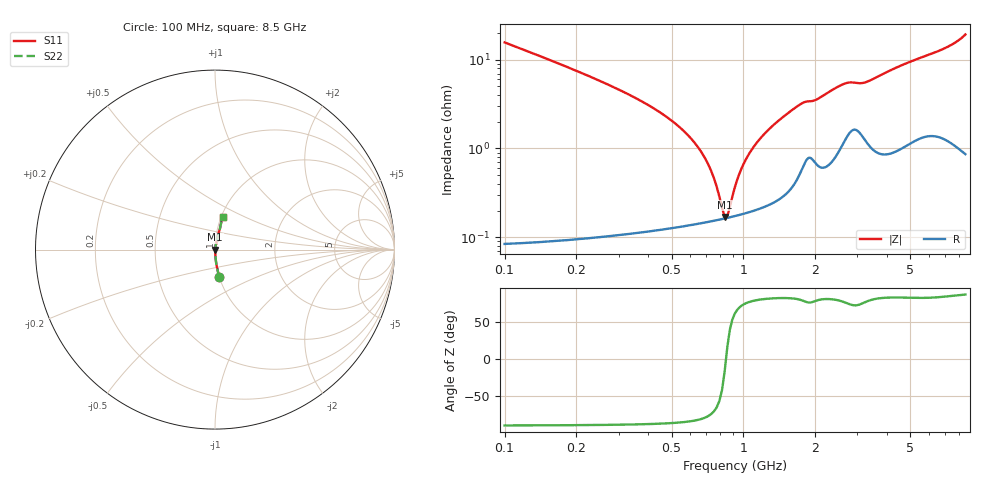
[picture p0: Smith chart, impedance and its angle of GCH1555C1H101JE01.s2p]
!Murata Part Number: GCH1555C1H101JE01
!These Parameters are Measured in Series Mode Connection
!Data Generated on Jun 19, 2026
!  o--ll--o
!Port1  Port2
!  o------o
!Operation Temp=25[degC], DC Bias Voltage=0[V]
!Freq. Start=100[MHz] Stop=9[GHz] 401[Steps]
# Hz S RI R 50
!Freq.(Hz) S11(Real) S11(Imag) S21(Real) S21(Imag) S12(Real) S12(Imag) S22(Real) S22(Imag)
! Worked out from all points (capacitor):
!   401 points, 100 MHz to 8.5 GHz, reference 50 ohm
!   read as one part in series: C = 100 pF near 142 MHz
!   lowest |Z| = 169 mohm at 835 MHz (marker M1)
!   series resonance near 845.3 MHz, so ESL is about 350 pH
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1e8  0.0248 -0.1528  0.9752 0.1528  0.9752 0.1528  0.0248 -0.1528
2.47e8  0.00443 -0.0585  0.9956 0.0585  0.9956 0.0585  0.00443 -0.0585
5.41e8  0.0016 -0.0172  0.9984 0.0172  0.9984 0.0172  0.0016 -0.0172
6.46e8  0.00152 -0.0102  0.9985 0.0102  0.9985 0.0102  0.00152 -0.0102
7.09e8  0.00153 -0.00661  0.9985 0.00661  0.9985 0.00661  0.00153 -0.00661
8.14e8  0.0016 -0.00141  0.9984 0.00141  0.9984 0.00141  0.0016 -0.00141
8.35e8  0.00163 -0.000457  0.9984 0.000457  0.9984 0.000457  0.00163 -0.000457
8.56e8  0.00165 0.000475  0.9984 -0.000475  0.9984 -0.000475  0.00165 0.000475
8.77e8  0.00168 0.00138  0.9983 -0.00138  0.9983 -0.00138  0.00168 0.00138
9.82e8  0.00184 0.00566  0.9982 -0.00566  0.9982 -0.00566  0.00184 0.00566
1.087e9  0.00205 0.0096  0.998 -0.0096  0.998 -0.0096  0.00205 0.0096
1.255e9  0.00249 0.0154  0.9975 -0.0154  0.9975 -0.0154  0.00249 0.0154
1.507e9  0.00362 0.0237  0.9964 -0.0237  0.9964 -0.0237  0.00362 0.0237
1.759e9  0.00681 0.0314  0.9932 -0.0314  0.9932 -0.0314  0.00681 0.0314
2.011e9  0.00789 0.0342  0.9921 -0.0342  0.9921 -0.0342  0.00789 0.0342
2.473e9  0.0109 0.0476  0.9891 -0.0476  0.9891 -0.0476  0.0109 0.0476
2.914e9  0.0187 0.0509  0.9813 -0.0509  0.9813 -0.0509  0.0187 0.0509
3.25e9  0.0148 0.053  0.9852 -0.053  0.9852 -0.053  0.0148 0.053
4.3e9  0.0152 0.0776  0.9848 -0.0776  0.9848 -0.0776  0.0152 0.0776
5.707e9  0.0243 0.104  0.9757 -0.104  0.9757 -0.104  0.0243 0.104
7.114e9  0.0301 0.1322  0.9699 -0.1322  0.9699 -0.1322  0.0301 0.1322
8.5e9  0.0434 0.1826  0.9566 -0.1826  0.9566 -0.1826  0.0434 0.1826
